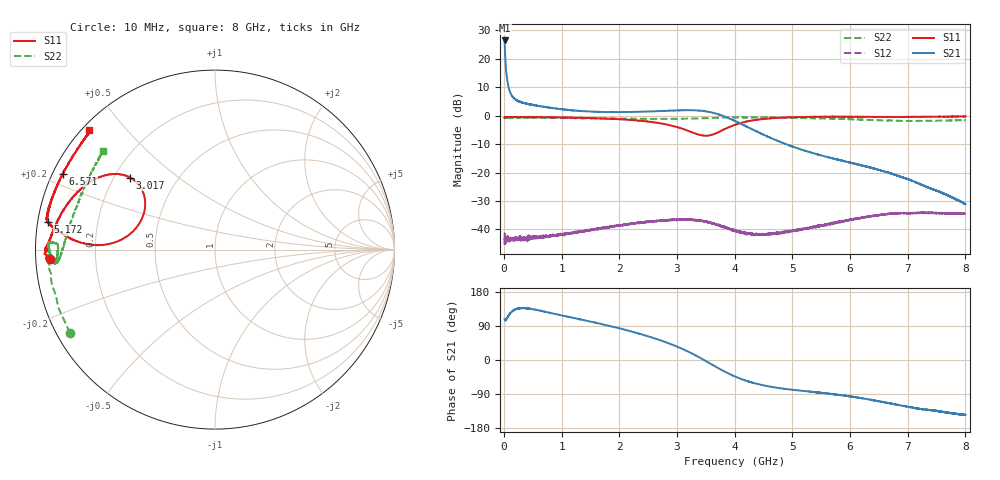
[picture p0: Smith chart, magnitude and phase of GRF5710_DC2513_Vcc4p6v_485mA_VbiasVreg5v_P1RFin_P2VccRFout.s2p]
!Keysight Technologies,N5244B,MY57181157,A.18.40.03
!Date: Thursday, September 18, 2025 15:48:54
!Correction: S11(C  2-Port  )
!S21(C  2-Port  )
!S12(C  2-Port  )
!S22(C  2-Port  )
!S2P File: Measurements: S11, S21, S12, S22:
# Hz S  RI  R 50
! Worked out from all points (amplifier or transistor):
!   7991 points, 10 MHz to 8 GHz, reference 50 ohm
!   highest |S21| = 26.4 dB at 10 MHz (marker M1)
!   |S21| within 3 dB of that: start of sweep to 14.23 MHz
!   unconditionally stable (mu >= 1): 122.6 MHz to 125.2 MHz; 126.4 MHz to 129.6 MHz; 132.1 MHz to end of sweep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
!   at 1.341 GHz: K = 1.93, MAG = 15.6 dB, |S12| = -40.7 dB
!   at 4.005 GHz: K = 5.58, MAG = 8.9 dB, |S12| = -40.5 dB
!   at 8 GHz: K = 17.35, MAG = -13.7 dB, |S12| = -34.5 dB
!   S11 on the Smith chart (normalised r, x): 10 MHz: 0.04, -0.03; 3.017 GHz: 0.26, +0.34; 5.172 GHz: 0.03, +0.08; 6.571 GHz: 0.03, +0.24; 8 GHz: 0.02, +0.40
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1e7  -0.918 -0.0541  -6.431 19.87  0.00583 0.00293  -0.8084 -0.4629
5e7  -0.937 -0.0103  -1.555 4.263  0.00649 0.000468  -0.9275 -0.0955
5.5e7  -0.9387 -0.00221  -1.501 3.857  0.00642 -0.000131  -0.9212 -0.0917
6.1e7  -0.9414 -0.0135  -1.544 3.527  0.00714 0.00107  -0.9275 -0.0856
7.4e7  -0.9394 -0.00485  -1.477 2.935  0.00679 0.000377  -0.9266 -0.0741
9.1e7  -0.9414 -0.00271  -1.428 2.438  0.00708 3.33e-05  -0.9265 -0.0605
1.13e8  -0.9399 0.00342  -1.368 2.035  0.0071 -0.000334  -0.9229 -0.0477
1.42e8  -0.9401 0.00166  -1.368 1.724  0.00684 0.000379  -0.9317 -0.0394
2.21e8  -0.9419 0.00581  -1.301 1.313  0.00658 0.000386  -0.9226 -0.0301
3.52e8  -0.94 0.00521  -1.211 1.131  0.00689 0.00113  -0.9272 -0.0359
1.342e9  -0.9089 0.0865  -0.341 1.152  0.00895 0.00217  -0.893 -0.0729
2.674e9  -0.6158 0.4132  0.7044 0.9659  0.0134 -0.00442  -0.8747 0.00471
3.017e9  -0.4731 0.4014  1.021 0.6945  0.0117 -0.00943  -0.876 0.0283
3.484e9  -0.4026 0.1838  1.192 -0.0306  0.00161 -0.0138  -0.8985 0.0391
3.753e9  -0.5299 0.0522  0.9303 -0.4265  -0.00561 -0.0101  -0.9167 0.0393
4.005e9  -0.6898 0.0271  0.5822 -0.5544  -0.00836 -0.00431  -0.9249 0.0389
4.465e9  -0.8592 0.0953  0.1969 -0.437  -0.00723 0.00354  -0.9264 0.00796
5.172e9  -0.9307 0.1544  0.0372 -0.2467  -0.00414 0.00917  -0.9034 -0.0614
5.337e9  -0.9378 0.1631  0.0235 -0.2213  -0.00358 0.0103  -0.897 -0.0711
6.571e9  -0.8479 0.4232  -0.038 -0.0993  0.00393 0.0174  -0.8157 0.1144
6.669e9  -0.8305 0.4536  -0.0402 -0.0908  0.00494 0.018  -0.8069 0.15
8e9  -0.7024 0.6663  -0.0229 -0.0162  0.0123 0.0143  -0.624 0.552
